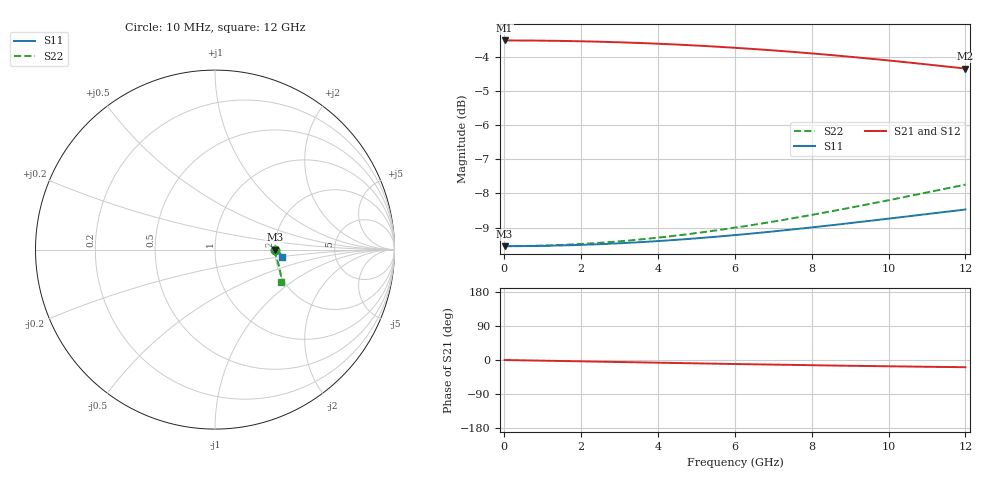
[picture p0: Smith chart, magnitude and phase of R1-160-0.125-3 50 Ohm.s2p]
!version-1
!date-03.2021
# MHz S RI R 50
!Freq ReS11 ImS11 ReS21 ImS21 ReS12 ImS12 ReS22 ImS22
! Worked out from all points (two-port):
!   601 points, 10 MHz to 12 GHz, reference 50 ohm
!   highest |S21| = -3.52 dB at 10 MHz (marker M1); lowest = -4.3 dB at 12 GHz (marker M2)
!   |S21| within 3 dB of the highest: start of sweep to end of sweep
!   lowest |S11| = -9.5 dB at 10 MHz (marker M3), VSWR 2.00, Z = 100 - j3.65e-05 ohm
!   |S11| at or under -10 dB: nowhere
!   |S22| runs from -9.5 to -7.7 dB; largest |S21 - S12| = 0
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10  0.3333 -1.62e-07  0.6667 -0.000211  0.6667 -0.000211  0.3333 -9.38e-05
70  0.3333 -1.14e-06  0.6667 -0.00148  0.6667 -0.00148  0.3333 -0.000657
1010  0.3337 -4.01e-05  0.6659 -0.0213  0.6659 -0.0213  0.3338 -0.00952
1510  0.3342 -0.000104  0.6649 -0.0318  0.6649 -0.0318  0.3344 -0.0143
2010  0.3348 -0.00022  0.6635 -0.0422  0.6635 -0.0422  0.3353 -0.0192
3010  0.3366 -0.00068  0.6596 -0.0627  0.6596 -0.0627  0.3376 -0.0294
4010  0.3391 -0.00156  0.6542 -0.0826  0.6542 -0.0826  0.3407 -0.0404
4990  0.3422 -0.00298  0.6475 -0.1014  0.6475 -0.1014  0.3444 -0.0521
6010  0.346 -0.00519  0.6393 -0.1198  0.6393 -0.1198  0.3487 -0.0655
6530  0.3481 -0.00665  0.6346 -0.1288  0.6346 -0.1288  0.351 -0.073
7030  0.3503 -0.00831  0.6298 -0.1371  0.6298 -0.1371  0.3533 -0.0805
7530  0.3526 -0.0102  0.6248 -0.145  0.6248 -0.145  0.3555 -0.0884
8010  0.3549 -0.0123  0.6197 -0.1523  0.6197 -0.1523  0.3577 -0.0964
8510  0.3574 -0.0148  0.6143 -0.1595  0.6143 -0.1595  0.3598 -0.1051
9010  0.3599 -0.0176  0.6086 -0.1663  0.6086 -0.1663  0.3619 -0.1143
9510  0.3624 -0.0208  0.6029 -0.1727  0.6029 -0.1727  0.3638 -0.124
10010  0.365 -0.0243  0.597 -0.1786  0.597 -0.1786  0.3654 -0.1341
10510  0.3675 -0.0281  0.5911 -0.1841  0.5911 -0.1841  0.3668 -0.1447
11030  0.3701 -0.0326  0.5848 -0.1893  0.5848 -0.1893  0.368 -0.1562
11570  0.3728 -0.0377  0.5784 -0.1942  0.5784 -0.1942  0.3688 -0.1687
11930  0.3745 -0.0414  0.5741 -0.1971  0.5741 -0.1971  0.369 -0.1773
12000  0.3748 -0.0421  0.5733 -0.1976  0.5733 -0.1976  0.369 -0.179
